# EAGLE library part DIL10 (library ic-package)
Dual In Line / Socket
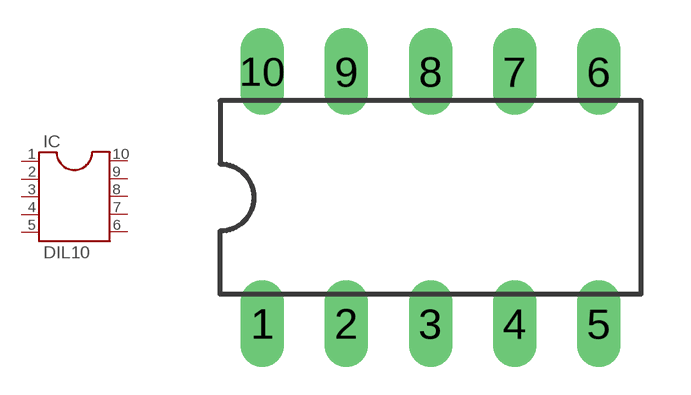
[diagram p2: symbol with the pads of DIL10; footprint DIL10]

Designator prefix IC

## DIL10  [DIL10]
1  1  pas
2  2  pas
3  3  pas
4  4  pas
5  5  pas
6  6  pas
7  7  pas
8  8  pas
9  9  pas
10  10  pas

## Footprint DIL10 (pad centres in mm)
Dual In Line Package
drill 0.813 long: 1 -5.08,-3.81; 2 -2.54,-3.81; 3 0,-3.81; 4 2.54,-3.81; 5 5.08,-3.81; 6 5.08,3.81; 7 2.54,3.81; 8 0,3.81; 9 -2.54,3.81; 10 -5.08,3.81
